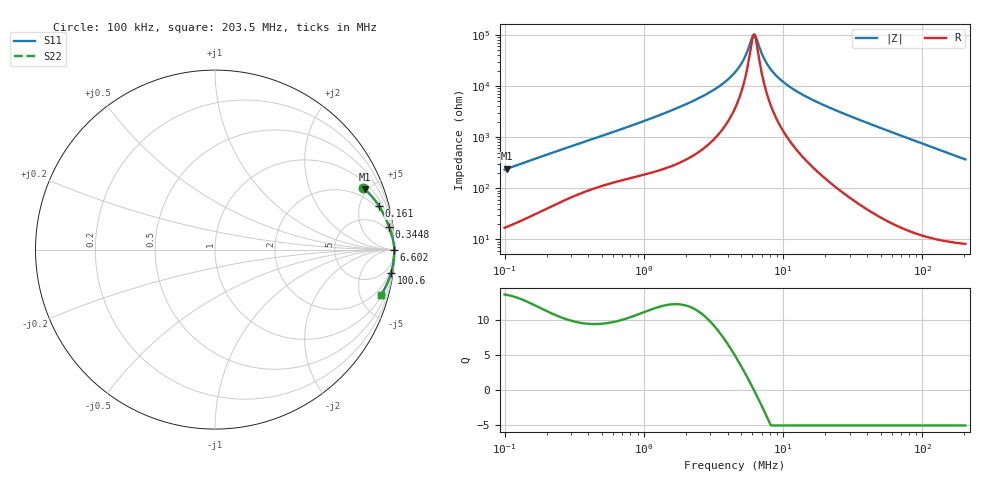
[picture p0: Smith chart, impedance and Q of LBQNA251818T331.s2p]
! LBQNA251818T331  S-PARAMETER MODEL  ( General Type )
! Model Generated by TAIYO YUDEN Corporation (http://www.ty-top.com)
! Version 1.0
! TAIYO YUDEN Control No. 191025NI43SB-FBB
! Copyright(c) 2019 TAIYO YUDEN CO.,LTD. All Rights Reserved.
! Product Description (link to TY-COMPAS)
! https://ds.yuden.co.jp/TYCOMPAS/or/detail?pn=LBQNA251818T331K&u=M
! Products Name : Inductors
! Characteristics :
!  Inductance : 330 uH , SRF(min) : 4.5 MHz , DC Resistance(max) : 9.1 Ohm
!  Rated Current : Saturation :40 mA , Temp Rise : 90 mA (20 degC)
!  Case Size : 2.5 x 1.8 / 0.098 x 0.071 [mm/inch] , Thickness : 1.8 / 0.071 [mm/inch]
!  (Conditions: Temperature = 25 degC , DC Bias Current/Voltage = 0A / 0V)
! External Node Assignments :
!  1  o---GGG---o  2
! GND o---------o GND
! Frequency Range : 0.1MHz  -  203.457813MHz  [ 402 STEP ]
# MHz S RI R 50
! Freq[MHz].  S11 Real  S11 Imag  S21 Real  S21 Imag  S12 Real  S12 Imag  S22 Real  S22 Imag
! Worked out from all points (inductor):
!   401 points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, 100 kHz to 203.5 MHz, reference 50 ohm
!   read as one part in series: L = 365 uH near 103.9 kHz
!   highest Q = 13.6 at 103.9 kHz (marker M1), where L = 367 uH
!   self-resonance near 6.118 MHz
!   S11 on the Smith chart (normalised r, x): 100 kHz: 1.34, +4.61; 161 kHz: 1.60, +7.32; 344.8 kHz: 3, +15; 6.602 MHz: open; 100.6 MHz: 1, -15; 203.5 MHz: 1.16, -7.32
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0.1  0.8251 0.345  0.1749 -0.345  0.1749 -0.345  0.8251 0.345
0.103882  0.8347 0.3365  0.1653 -0.3365  0.1653 -0.3365  0.8347 0.3365
0.160983  0.9139 0.2425  0.0861 -0.2425  0.0861 -0.2425  0.9139 0.2425
0.344848  0.9699 0.1266  0.0301 -0.1266  0.0301 -0.1266  0.9699 0.1266
0.358236  0.9714 0.1224  0.0286 -0.1224  0.0286 -0.1224  0.9714 0.1224
1.283332  0.9955 0.0372  0.00454 -0.0372  0.00454 -0.0372  0.9955 0.0372
2.910717  0.9985 0.0136  0.00155 -0.0136  0.00155 -0.0136  0.9985 0.0136
3.728424  0.9988 0.00873  0.00124 -0.00873  0.00124 -0.00873  0.9988 0.00873
4.51063  0.9989 0.00531  0.0011 -0.00531  0.0011 -0.00531  0.9989 0.00531
5.153894  0.999 0.00303  0.00103 -0.00303  0.00103 -0.00303  0.999 0.00303
5.456938  0.999 0.00208  0.00101 -0.00208  0.00101 -0.00208  0.999 0.00208
5.888895  0.999 0.000808  0.000989 -0.000808  0.000989 -0.000808  0.999 0.000808
6.117531  0.999 0.000177  0.000979 -0.000177  0.000979 -0.000177  0.999 0.000177
6.355044  0.999 -0.000455  0.000972 0.000455  0.000972 0.000455  0.999 -0.000455
6.601778  0.999 -0.00109  0.000965 0.00109  0.000965 0.00109  0.999 -0.00109
7.400959  0.999 -0.003  0.000954 0.003  0.000954 0.003  0.999 -0.003
8.784736  0.999 -0.00595  0.00096 0.00595  0.00096 0.00595  0.999 -0.00595
11.25263  0.999 -0.0105  0.00102 0.0105  0.00102 0.0105  0.999 -0.0105
16.15871  0.9987 -0.0185  0.00125 0.0185  0.00125 0.0185  0.9987 -0.0185
57.88634  0.9929 -0.0763  0.00714 0.0763  0.00714 0.0763  0.9929 -0.0763
100.5635  0.9802 -0.1317  0.0198 0.1317  0.0198 0.1317  0.9802 -0.1317
203.4578  0.9257 -0.2514  0.0743 0.2514  0.0743 0.2514  0.9257 -0.2514
